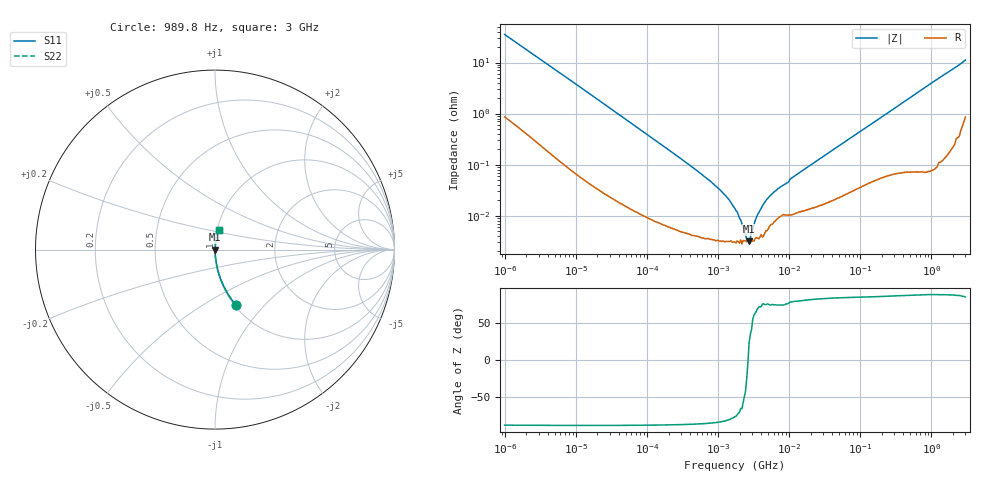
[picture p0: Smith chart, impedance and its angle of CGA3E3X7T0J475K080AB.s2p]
! S-Parameter Data Generated by TDK Corporation
! Copyright(C) 2024 TDK Corporation.
! All Rights Reserved.
! TDK P/N: CGA3E3X7T0J475K080AB (Multilayer Ceramic Chip Capacitor)
! Property: C=4.7uF
! Size(LxWxT): 1.6x0.8x0.8mm
! Model Type: s2p (Touchstone File Format Version 1.0)
! Frequency: DC=Yes Start=0.000989846MHz Stop=3000MHz 523points Log-sweep
! Model Generated on May 28, 2024
! Terms and conditions regarding TDK Simulation Models:
! 1)This simulation model is being provided solely for informational
!  purposes. Please refer to the specifications of the products in
!  terms of detailed characteristics of such products.
! 2)In no event shall TDK Corporation of any of its subsidiaries be
!  liable for any loss or damage arising, directly or indirectly,
!  from any information contained in this simulation model, including,
!  but not limited to loss or damages arising from any inaccuracies,
!  omissions or errors in connection with such information.
! 3)Any and all copyrights on this simulation model are owned by
!  TDK Corporation.  Duplication or redistribution of this simulation
!  model without prior written permission from TDK Corporation
!  is prohibited.
! 4)This simulation model is subject to any modification or change
!  without any prior notice.
! 5)Neither TDK Corporation nor any of its subsidiaries shall make any
!  warranty, express or implied, including but not limited to the
!  correctness, implied warranties of merchantability and fitness for
!  a particular purpose with respect to this simulation models.
! 6)The use of this simulation model shall be deemed to have consented
!  to the terms and conditions hereof.
! Port Assignments:
!  1 ---| |--- 2
! Applicable Conditions:
!  Temperature = 25 degC
!  DC Bias Voltage = 0 V
!  Small Signal Operation
# Hz S MA R 50
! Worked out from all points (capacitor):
!   522 points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, 989.8 Hz to 3 GHz, reference 50 ohm
!   read as one part in series: C = 4.5 uF near 1.07 kHz
!   lowest |Z| = 3.13 mohm at 2.726 MHz (marker M1)
!   series resonance near 2.633 MHz, so ESL is about 810 pH
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989.846  0.332 -69.2  0.9353 19.4  0.9353 19.4  0.332 -69.2
1643.83  0.2109 -76.5  0.9727 12.2  0.9727 12.2  0.2109 -76.5
3068.91  0.1175 -82.1  0.9906 6.7  0.9906 6.7  0.1175 -82.1
12024.6  0.03143 -87.2  0.999 1.8  0.999 1.8  0.03143 -87.2
146075  0.002674 -88.3  0.9999 0.2  0.9999 0.2  0.002674 -88.3
452889  0.0008525 -87.2  1 0.0  1 0.0  0.0008525 -87.2
845509  0.0004259 -85.5  1 0.0  1 0.0  0.0004259 -85.5
1298730  0.0002378 -82.4  1 0.0  1 0.0  0.0002378 -82.4
1774520  0.0001265 -76.7  1 0.0  1 0.0  0.0001265 -76.7
2074250  8.211e-05 -65.9  1 0.0  1 0.0  8.211e-05 -65.9
2725710  3.13e-05 23.9  1 -0.0  1 -0.0  3.13e-05 23.9
3444700  9.195e-05 66.3  1 -0.0  1 -0.0  9.195e-05 66.3
3724280  0.0001143 72.1  1 -0.0  1 -0.0  0.0001143 72.1
4706680  0.0001995 75.2  0.9999 -0.0  0.9999 -0.0  0.0001995 75.2
5720600  0.0002665 75.4  0.9999 -0.0  0.9999 -0.0  0.0002665 75.4
7229600  0.0003493 74.6  0.9999 -0.0  0.9999 -0.0  0.0003493 74.6
9136640  0.0004312 76.1  0.9999 -0.0  0.9999 -0.0  0.0004312 76.1
1.06109e7  0.0005356 78.8  0.9999 -0.0  0.9999 -0.0  0.0005356 78.8
2.09559e7  0.001029 82.1  0.9999 -0.1  0.9999 -0.1  0.001029 82.1
2.50734e8  0.01063 86.1  0.9993 -0.6  0.9993 -0.6  0.01063 86.1
1.05949e9  0.04183 86.5  0.9983 -2.4  0.9983 -2.4  0.04183 86.5
3e9  0.1101 79.3  0.9855 -6.3  0.9855 -6.3  0.1101 79.3
